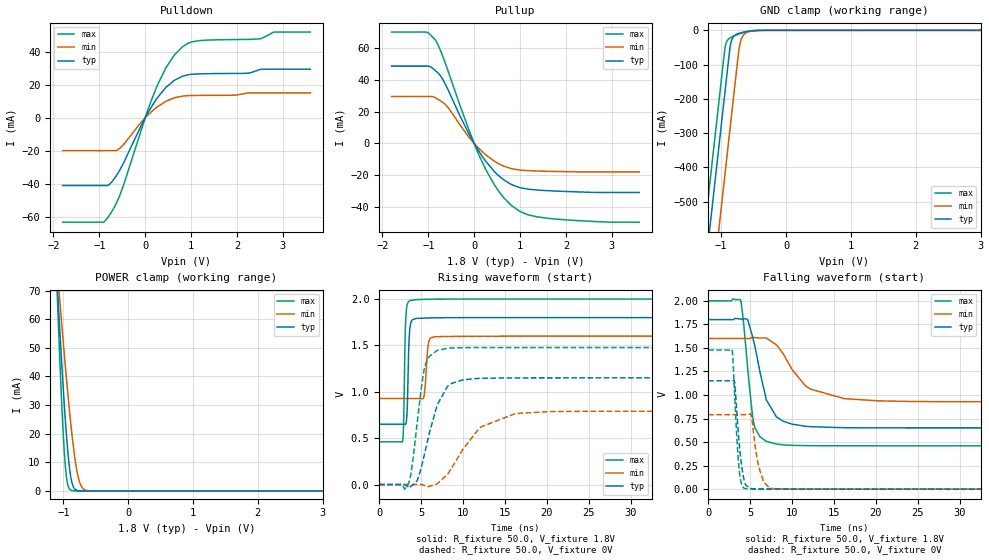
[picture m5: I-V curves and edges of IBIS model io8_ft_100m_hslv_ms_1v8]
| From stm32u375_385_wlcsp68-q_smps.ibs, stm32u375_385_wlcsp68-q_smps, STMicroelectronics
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[Model]   io8_ft_100m_hslv_ms_1v8
Model_type I/O
Polarity   Non-Inverting
Enable   Active-Low
| CAP_THRESHOLD on pad IOFT is "UDTCAPC" :
| Rising=30.0% of vddiom   Falling=70.0% of vddiom
| C_comp min and max val. don't necessarily correlate with the min and max pvt
| but are the smallest and greatest pad capacitance found.
| var   typ   min   max
C_comp   3.41787pF  3.41663pF  3.48192pF
|C_comp_pullup   1.92549pF  1.84320pF  2.10227pF
|C_comp_pulldown   1.49238pF  1.57343pF  1.37964pF
Vinl = 800.0mV
Vinh = 1.0V
Vmeas = 900.0mV   | Reference voltage for timing measurements
Cref  = 50.0pF   | Timing specification test load capacitance value
Rref  = 1.0MOhm   | Timing specification test load resistance value
Vref  = 990.0mV   | Timing specification test load voltage
[Model Spec]
| TIME_THRESHOLD on pin ZIV11 is "CMOS" :
| Rising=50.0% of vdd   Falling=50.0% of vdd
Vinl 694.50000mV 619.50000mV 778.50000mV
Vinh 1.08350V 957.50000mV 1.18750V
| variable   typ   min   max
[Temperature Range] 25.0 130.0 -40.0
| variable   typ   min   max
[Voltage Range] 1.8V 1.6V 2.0V
| variable   typ   min   max
[POWER Clamp Reference] 1.8V 1.6V 2.0V
| variable   typ   min   max
[GND Clamp Reference] 0V 0V 0V
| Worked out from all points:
|   slope of the pulldown table from 0 to 0.27 V, typ, clamps not added: 21.9 ohm
|   slope of the pullup table from 0 to 0.27 V, typ, clamps not added: 22.8 ohm
|   GND clamp passes 1 mA (typ) near -0.50 V on its own axis
|   POWER clamp passes 1 mA (typ) near -0.83 V on its own axis
|   rising waveform, R_fixture 50.0, V_fixture 1.8V: 20-80 % time 205ps typ, 302ps min, 193ps max; typ from 0.65 V to 1.8 V
|   falling waveform, R_fixture 50.0, V_fixture 1.8V: 20-80 % time 1.96ns typ, 3.48ns min, 1.01ns max; typ from 1.8 V to 0.65 V
|   rising waveform, R_fixture 50.0, V_fixture 0V: 20-80 % time 2.15ns typ, 3.97ns min, 1.19ns max; typ from 0 V to 1.15 V
|   falling waveform, R_fixture 50.0, V_fixture 0V: 20-80 % time 686ps typ, 943ps min, 550ps max; typ from 1.15 V to 0 V
[POWER Clamp]
-1.8V     399.1mA    292.1mA    557.7mA
-1.09V    71.2mA     76.8mA     67.14mA
-1.08V    67.05mA    73.98mA    61.2mA
-1.06V    58.89mA    68.38mA    49.67mA
-1.02V    43.22mA    57.4mA     28.67mA
-980mV    28.81mA    46.77mA    12.28mA
-940mV    16.45mA    36.61mA    3.257mA
-880mV    4.35mA     22.67mA    225.4uA
-820mV    610.4uA    11.29mA    13uA
-770mV    97.5uA     4.87mA     1.193uA
-640mV    753.9nA    196uA      2.492nA
3.6V      0A         0A         0A
[GND Clamp]
-1.8V     -1.64A     -1.88A     -1.509A
-1.24V    -688.2mA   -927.9mA   -557mA
-1.05V    -365.2mA   -604.9mA   -234mA
-950mV    -195.2mA   -434.9mA   -64mA
-930mV    -161.2mA   -400.9mA   -41.59mA
-870mV    -59.19mA   -298.9mA   -22.94mA
-850mV    -36.73mA   -264.9mA   -20.65mA
-770mV    -12.21mA   -128.9mA   -13.73mA
-730mV    -9.139mA   -62.1mA    -10.81mA
-690mV    -6.97mA    -26.33mA   -8.198mA
-530mV    -1.564mA   -2.413mA   -1.407mA
3.6V      1.228nA    159.5nA    526.9pA
| variable   typ   min   max
[Pullup Reference] 1.8V 1.6V 2.0V
| variable   typ   min   max
[Pulldown Reference] 0V 0V 0V
[Pullup]
-1.8V     48.6mA     29.46mA    69.97mA
-1.04V    48.6mA     29.46mA    69.94mA
-840mV    45.64mA    28.62mA    64.71mA
-730mV    42.3mA     26.68mA    58.03mA
-590mV    34.96mA    23.2mA     47.23mA
-120mV    6.328mA    4.158mA    8.961mA
120mV     -5.719mA   -3.668mA   -8.284mA
440mV     -17.67mA   -11.15mA   -25.97mA
810mV     -25.79mA   -15.81mA   -38.95mA
1.18V     -28.75mA   -17.1mA    -44.89mA
1.56V     -29.61mA   -17.45mA   -46.86mA
3.6V      -30.8mA    -17.88mA   -49.48mA
[Pulldown]
-1.8V     -41.16mA   -19.96mA   -63.43mA
-920mV    -41.16mA   -19.96mA   -63.43mA
-780mV    -40.43mA   -19.96mA   -59.18mA
-510mV    -29.46mA   -17.38mA   -43.8mA
0V        0A         -230fA     0A
250mV     11.64mA    6.428mA    18.87mA
460mV     18.67mA    10.12mA    30.76mA
810mV     25.21mA    13.14mA    43.03mA
1.18V     26.67mA    13.59mA    46.9mA
2.5V      29.31mA    15.12mA    47.95mA
2.81V     29.55mA    15.12mA    52.03mA
3.6V      29.55mA    15.12mA    52.05mA
[Ramp]
dV/dt_r 690.02818mV/2.01534ns 474.37159mV/3.82863ns 886.36799mV/1.19311ns
dV/dt_f 689.75444mV/1.80825ns 402.99702mV/3.45853ns 923.68055mV/1.00866ns
R_load = 50.0
| Removed startup time: 0s 0s 0s  .
| Removed end time: 36.25ns.
[Rising Waveform]
R_fixture   = 50.0
V_fixture   = 1.8V
V_fixture_min = 1.6V
V_fixture_max = 2.0V
0s        650.4mV    928.3mV    460.5mV
2.8ns     650.6mV    928.3mV    473.9mV
2.9ns     650.6mV    928.3mV    632.7mV
3.15ns    650.3mV    928.3mV    1.764V
3.35ns    840mV      928.3mV    1.943V
3.65ns    1.679V     928.3mV    1.983V
5.3ns     1.795V     941.3mV    1.997V
5.85ns    1.796V     1.511V     1.998V
6.65ns    1.798V     1.593V     1.999V
36.25ns   1.8V       1.6V       2V
| Removed startup time: 0s 0s 0s  .
| Removed end time: 199.25ns.
[Falling Waveform]
R_fixture   = 50.0
V_fixture   = 1.8V
V_fixture_min = 1.6V
V_fixture_max = 2.0V
0s        1.8V       1.6V       2V
3.85ns    1.807V     1.6V       2.009V
4.7ns     1.797V     1.6V       1.293V
5.25ns    1.632V     1.61V      807.8mV
5.55ns    1.525V     1.609V     661.2mV
6.95ns    944.9mV    1.605V     507.6mV
8.95ns    721.7mV    1.438V     470.8mV
12.2ns    663.5mV    1.062V     461.6mV
20.35ns   650.7mV    937.3mV    460.5mV
199.3ns   650.4mV    928.3mV    460.5mV
| Removed startup time: 0s 0s 0s  .
| Removed end time: 199.2ns.
[Rising Waveform]
R_fixture   = 50.0
V_fixture   = 0V
V_fixture_min = 0V
V_fixture_max = 0V
0s        4.628nV    97.71nV    3.406nV
3.45ns    -27.67mV   -2.735uV   5.981mV
3.9ns     -11.39mV   -6.828uV   187.5mV
4.55ns    50.29mV    -54.28uV   685.2mV
5.5ns     367.9mV    -12.8mV    1.29V
6.9ns     856.4mV    7.387mV    1.446V
8.15ns    1.06V      109.7mV    1.469V
12.2ns    1.146V     623.2mV    1.477V
20.35ns   1.15V      786.6mV    1.477V
199.2ns   1.15V      790.6mV    1.477V
| Removed startup time: 0s 0s 0s  .
| Removed end time: 36.25ns.
[Falling Waveform]
R_fixture   = 50.0
V_fixture   = 0V
V_fixture_min = 0V
V_fixture_max = 0V
0s        1.15V      790.6mV    1.477V
2.85ns    1.15V      790.6mV    1.482V
3.15ns    1.138V     790.6mV    1.006V
3.65ns    537.3mV    790.6mV    248.9mV
3.9ns     314.7mV    790.7mV    81.39mV
4.3ns     90.51mV    790.7mV    9.782mV
5.1ns     6.807mV    793.5mV    2.043mV
6.15ns    2.076mV    200.7mV    1.075mV
7.4ns     1.101mV    9.215mV    503.3uV
36.25ns   59.05nV    751.7nV    8.161nV
